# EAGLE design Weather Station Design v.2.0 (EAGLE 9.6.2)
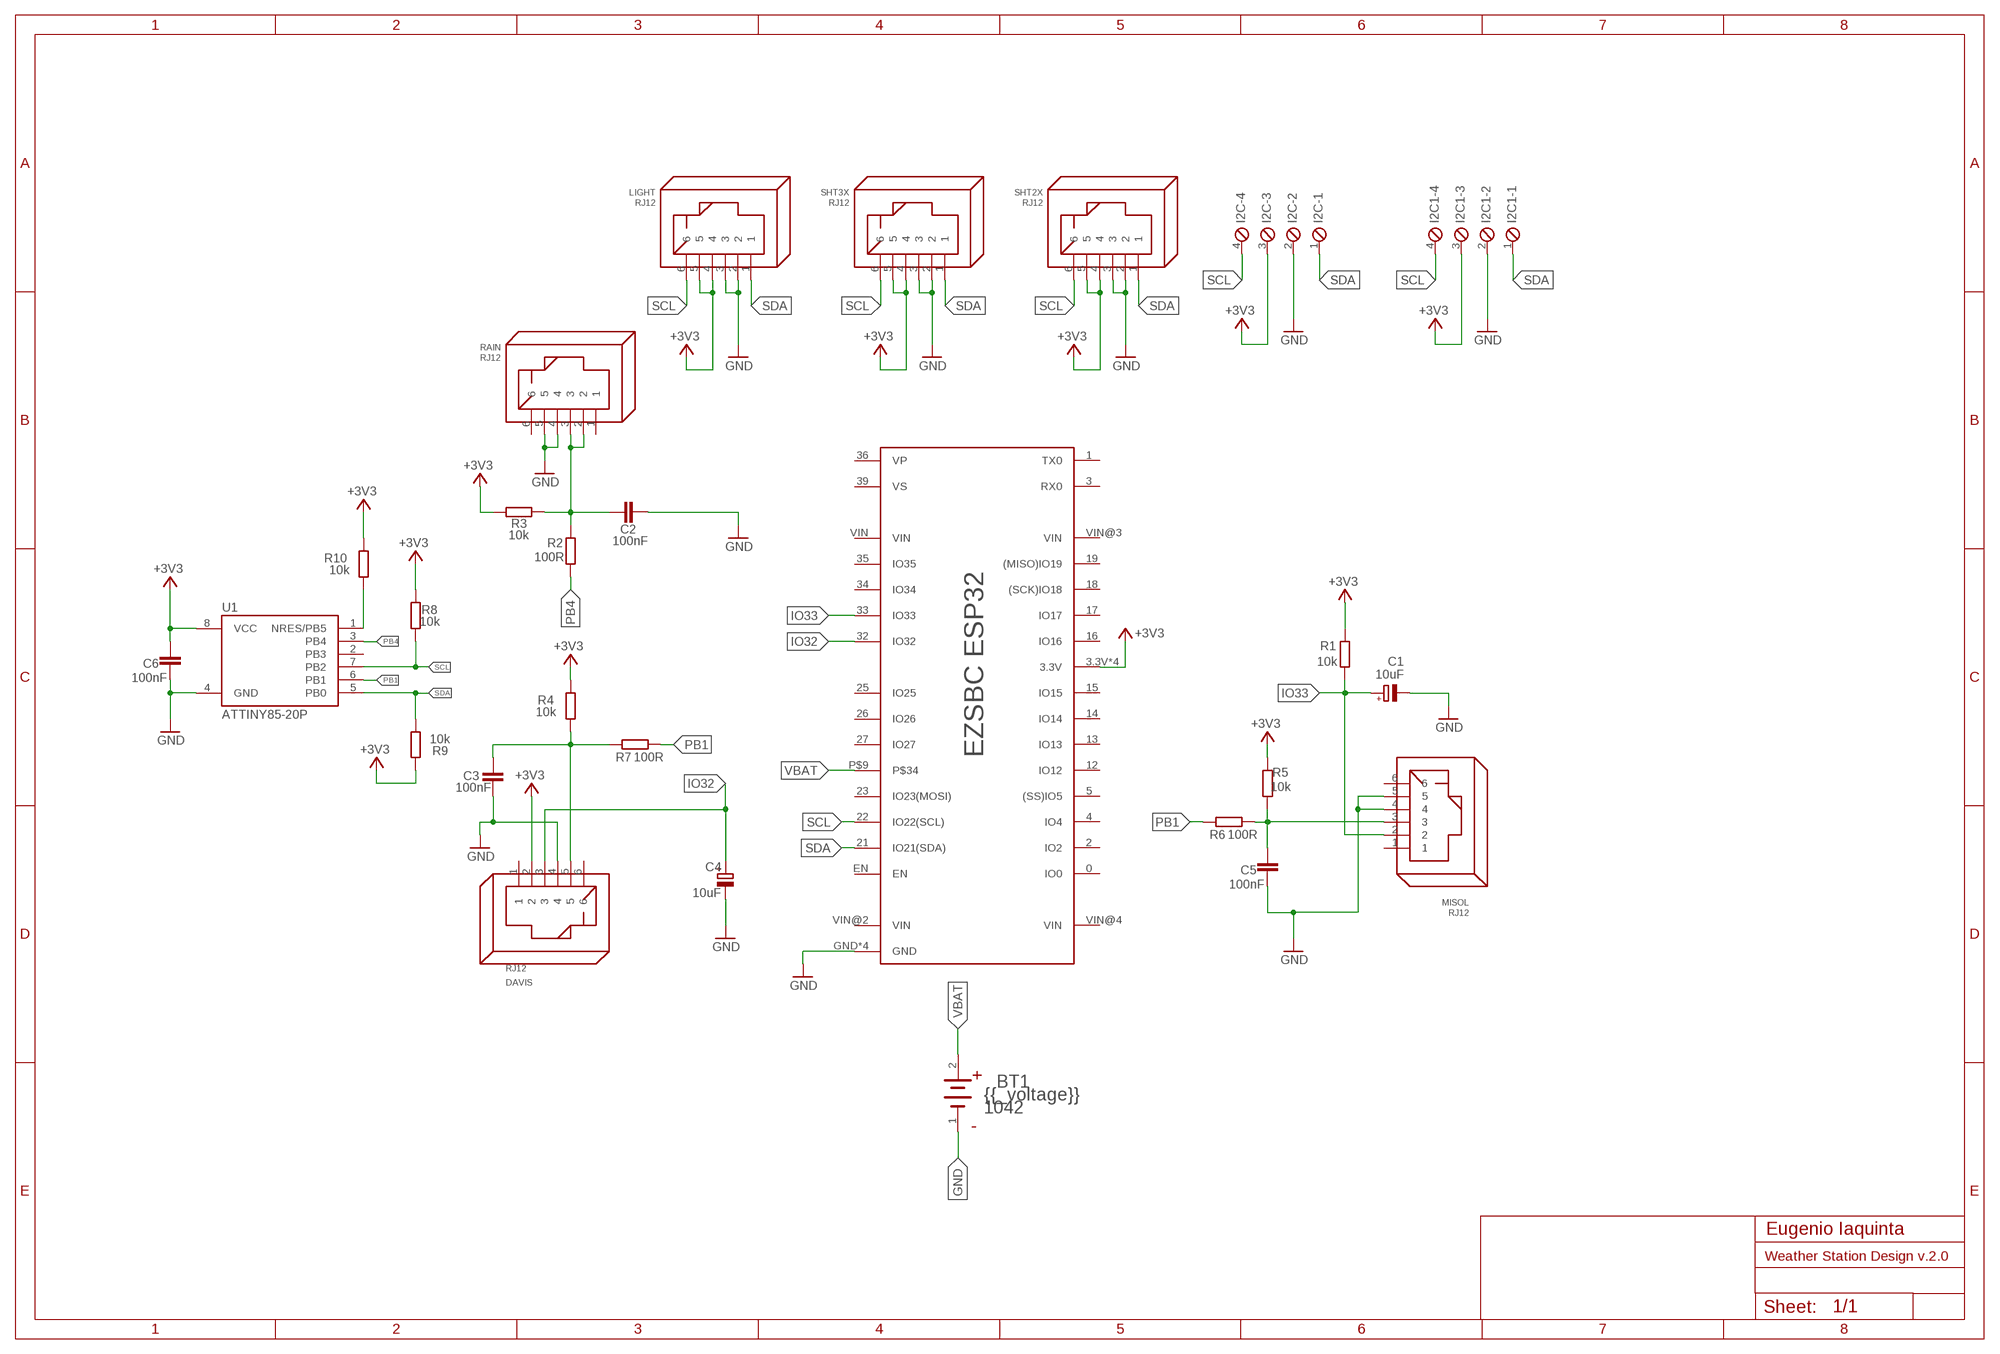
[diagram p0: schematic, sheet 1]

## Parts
BT1  KEYSTONE_1042KEYSTONE_1042_0_0  [KEYSTONE_1042_0]
C1  10uF  CPOL-EUE2.5-5  [E2,5-5]
C2  100nF  C-EUC0805  [C0805]
C3  100nF  C-EUC0805  [C0805]
C4  10uF  CPOL-EUE2.5-5  [E2,5-5]
C5  100nF  C-EUC0805  [C0805]
C6  100nF  C-EUC0805  [C0805]
DAVIS  RJ12  [RJ12]
I2C  MPT4  [4POL254]
I2C1  MPT4  [4POL254]
LIGHT  RJ12  [RJ12]
MISOL  RJ12  [RJ12]
R1  10k  R-EU_M0805  [M0805]
R2  100R  R-EU_M0805  [M0805]
R3  10k  R-EU_M0805  [M0805]
R4  10k  R-EU_M0805  [M0805]
R5  10k  R-EU_M0805  [M0805]
R6  100R  R-EU_M0805  [M0805]
R7  100R  R-EU_M0805  [M0805]
R8  10k  R-EU_M0805  [M0805]
R9  10k  R-EU_M0805  [M0805]
R10  10k  R-EU_M0805  [M0805]
RAIN  RJ12  [RJ12]
SHT2X  RJ12  [RJ12]
SHT3X  RJ12  [RJ12]
U1  ATTINY85-20P  [PDIP08_300MIL]
U$1  EZSBCESP32  [EZSBCBATPRO]

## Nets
+3V3: C6.2 DAVIS.2 I2C1.3 I2C.3 LIGHT.4 LIGHT.5 R1.2 R3.1 R4.2 R5.2 R8.2 R9.2 R10.2 SHT2X.4 SHT2X.5 SHT3X.4 SHT3X.5 U1.8(VCC) U$1.3.3V U$1.3.3V@2(3.3V) U$1.3.3V@4(3.3V) U$1.3.3V@5(3.3V)
GND: BT1.1(CATHODE) C1.- C2.2 C3.2 C4.- C5.1 C6.1 DAVIS.4 I2C1.2 I2C.2 LIGHT.2 LIGHT.3 MISOL.4 MISOL.5 RAIN.4 RAIN.5 SHT2X.2 SHT2X.3 SHT3X.2 SHT3X.3 U1.4(GND) U$1.GND U$1.GND@2(GND) U$1.GND@3(GND) U$1.GND@4(GND)
IO32: C4.+ DAVIS.3 U$1.32(IO32)
IO33: C1.+ MISOL.2 R1.1 U$1.33(IO33)
N$4: C2.1 R2.2 R3.2 RAIN.2 RAIN.3
N$7: R10.1 U1.1(NRES/PB5)
PB1: R6.2 R7.1 U1.6(PB1)
PB4: R2.1 U1.3(PB4)
PIN3: C5.2 MISOL.3 R5.1 R6.1
PIN5: C3.1 DAVIS.5 R4.1 R7.2
SCL: I2C1.4 I2C.4 LIGHT.6 R8.1 SHT2X.6 SHT3X.6 U1.7(PB2) U$1.22(IO22(SCL))
SDA: I2C1.1 I2C.1 LIGHT.1 R9.1 SHT2X.1 SHT3X.1 U1.5(PB0) U$1.21(IO21(SDA))
VBAT: BT1.2(ANODE) U$1.P$9
Unconnected: DAVIS.1 DAVIS.6 MISOL.1 MISOL.6 RAIN.1 RAIN.6 U1.2(PB3) U$1.0(IO0) U$1.1(TX0) U$1.2(IO2) U$1.3(RX0) U$1.4(IO4) U$1.5((SS)IO5) U$1.12(IO12) U$1.13(IO13) U$1.14(IO14) U$1.15(IO15) U$1.16(IO16) U$1.17(IO17) U$1.18((SCK)IO18) U$1.19((MISO)IO19) U$1.23(IO23(MOSI)) U$1.25(IO25) U$1.26(IO26) U$1.27(IO27) U$1.34(IO34) U$1.35(IO35) U$1.36(VP) U$1.39(VS) U$1.EN U$1.VIN U$1.VIN@2(VIN) U$1.VIN@3(VIN) U$1.VIN@4(VIN)

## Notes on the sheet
- Eugenio Iaquinta

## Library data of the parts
BT1 = Keystone - 1042:KEYSTONE_1042: PC BATTERY HOLDER 18650; CENTROID_NOT_SPECIFIED: No; DATASHEET: http://www.keyelco.com/product-pdf.cfm?p=918; DIGIKEY_DESCRIPTION: BATT HOLDER BATTERY 1CELL 18650 SMD; DIGIKEY_PART_NUMBER: 36-1042-ND; IPC_LAND_PATTERN_NAME: CAPC200125X45; LEAD_FREE: yes; MF: Keystone; MOUSER_PART_NUMBER: 534-1042; MPN: 1042; PACKAGE: PTH_BAT_HOLDER_18650; PREFIX: BT; ROHS: yes
C1 C4 = rcl:CPOL-EU: POLARIZED CAPACITOR, European symbol; SPICEPREFIX: C
C2 C3 C5 C6 = rcl:C-EU: CAPACITOR, European symbol; SPICEPREFIX: C
DAVIS LIGHT MISOL RAIN SHT2X SHT3X = con-rj:RJ12: RJ12, RJ14 and RJ25 RJ12, RJ14 and RJ25 jacks side mounted http://www.tycoelectronics.com
I2C I2C1 = con-phoenix-254:MPT4: PHOENIX CONNECTOR; OC_FARNELL: unknown; OC_NEWARK: unknown
R1-R10 = rcl:R-EU_: RESISTOR, European symbol; SPICEPREFIX: R
U1 = attiny25_45_85:ATTINY85*: ATMEL ATtiny 85 Packages: P = PDIP 08 30mil S = SOIC 08 EIAJ 208mil Technologies Note: for complete ordering code (temp. range, finish, tape&reel etc.) see www.atmel.com &bull; Supply Voltage: V = (1.8&hellip;5.5)V | [blank] = (2.7&hellip;5.5)V &bull; Speed: 10 = 10 MHz | 20 = 20 MHz Author: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
U$1 = EzbscBatESP32:EZSBCESP32

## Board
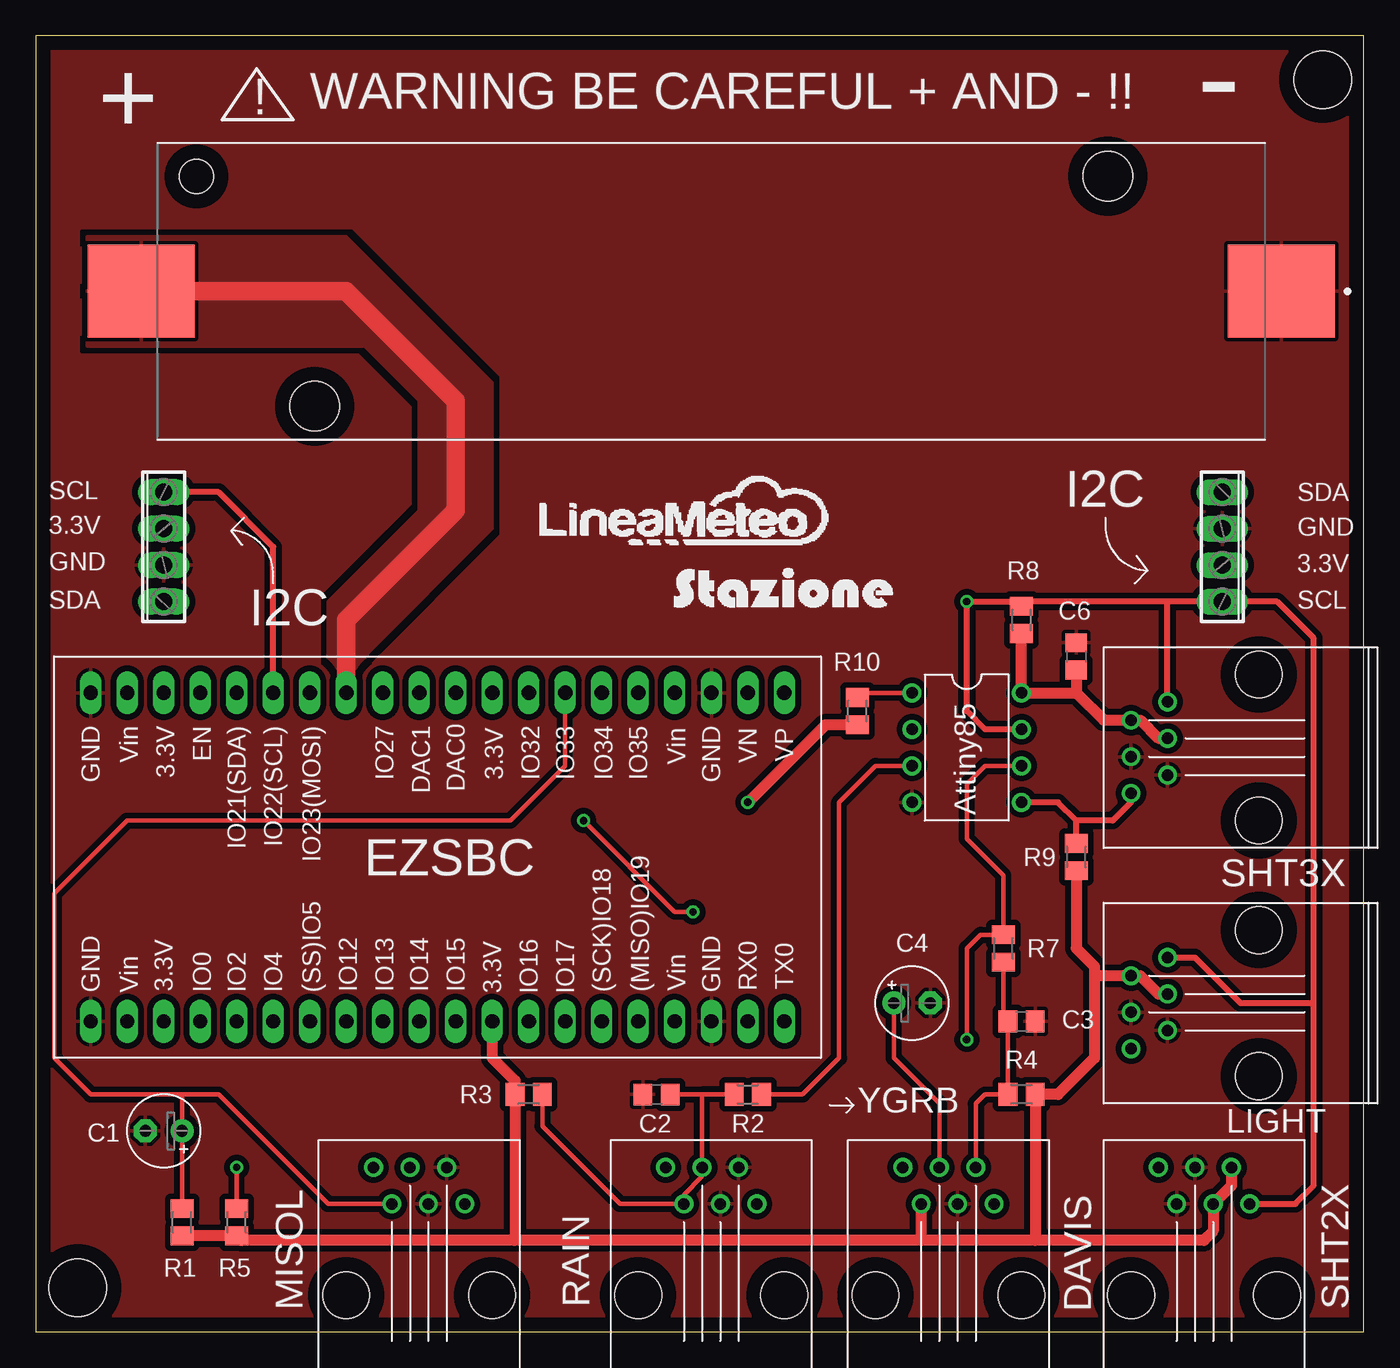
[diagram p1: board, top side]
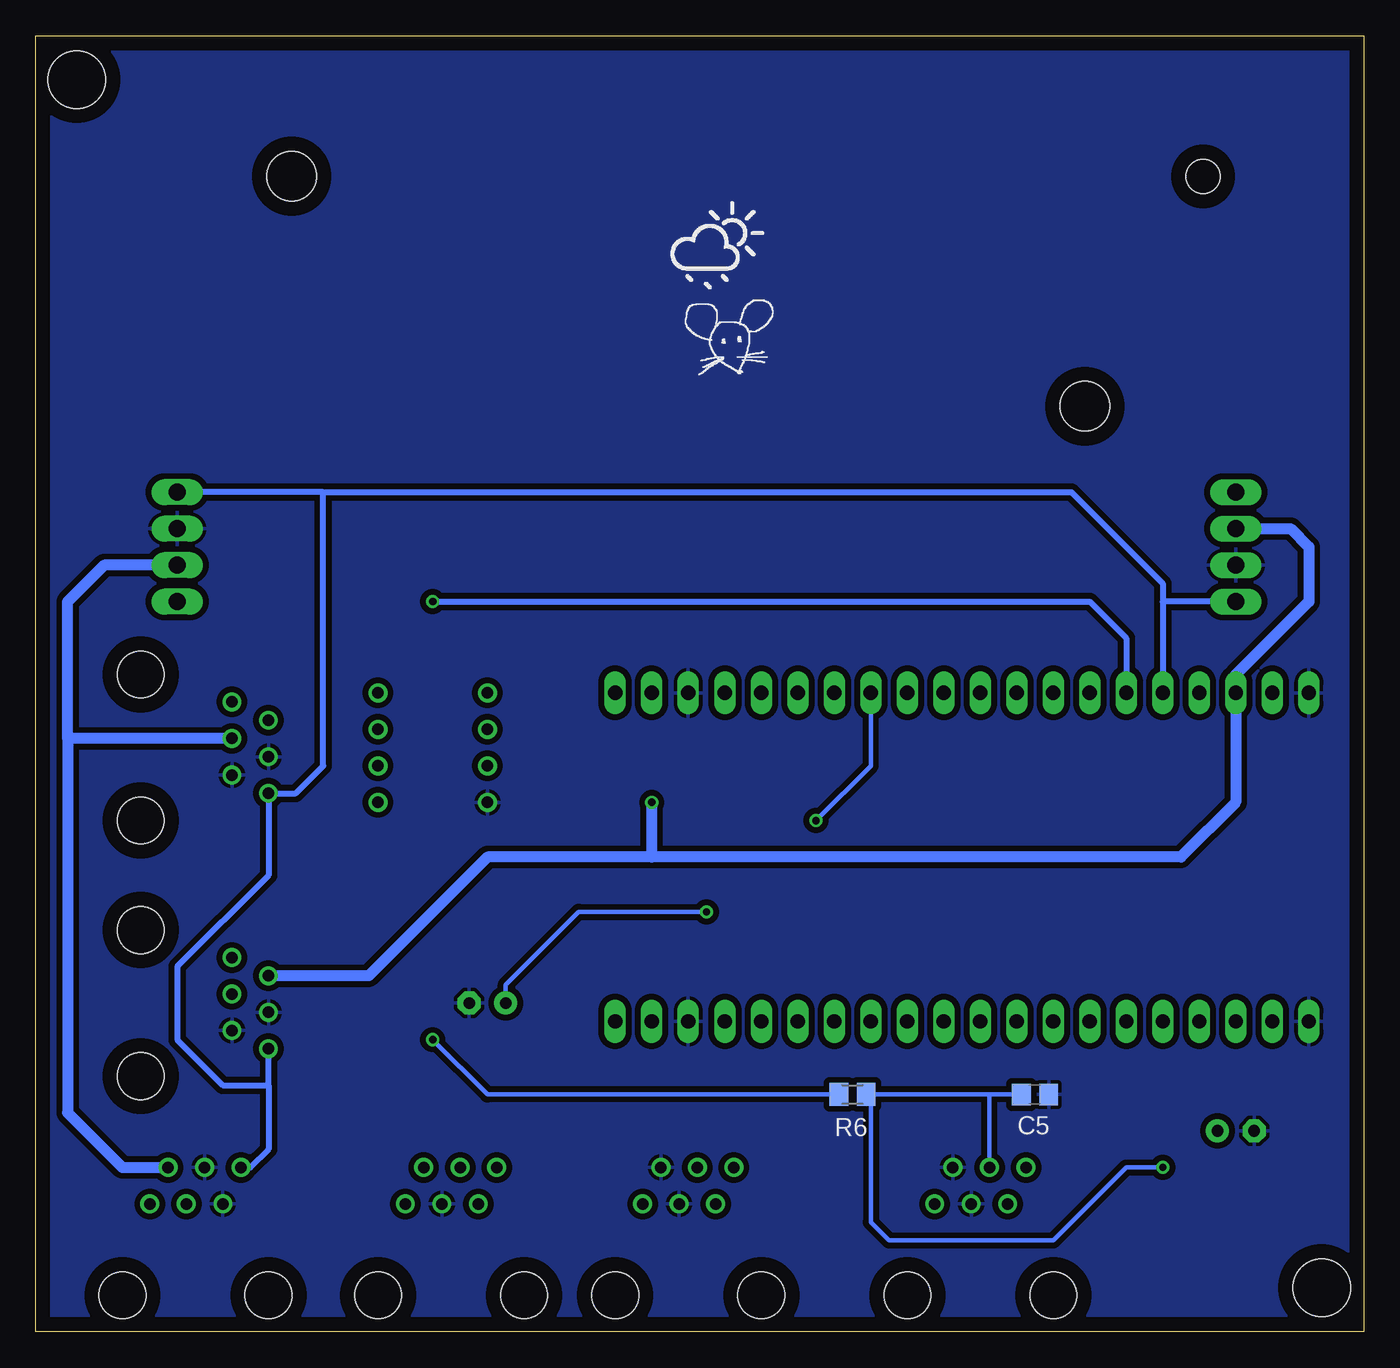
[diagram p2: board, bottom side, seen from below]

Size 92.38 x 90.16 mm. Coordinates in mm from the lower left corner, seen from the top.
Outline: 0,0 92.38,0 92.38,90.16 0,90.16 0,0
Copper layers (1*16): Top 0.035mm / dielectric 1.5mm / Bottom 0.035mm
Design rules "default": minimum track width 6mil, minimum drill 0.35mm, track to track 6mil, track to pad 6mil, pad to pad 6mil, via to via 6mil, smd to smd 6mil, copper to edge 40mil, drill to drill 6mil, minimum pad ring 10mil, minimum via ring 8mil, stop-mask expansion 4mil, vias tented up to drill 0mil, thermal gap 10mil
Holes 4 mm at 89.53,87.12 2.92,3.05

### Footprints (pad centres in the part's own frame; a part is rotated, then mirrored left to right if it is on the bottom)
KEYSTONE_1042_0 = smd 7.46 x 6.47: 1 -39.67,0; 2 39.67,0 | hole 3.45: -27.6,-8; 27.6,8 | hole 2.39: 35.82,-8
E2,5-5 = drill 0.813 pad 1.6: + -1.27,0 | drill 0.813 pad 1.6 octagon: - 1.27,0
C0805 = smd 1.3 x 1.5: 1 -0.95,0; 2 0.95,0
RJ12 = drill 0.8: 1 -8.89,-3.175; 2 -6.35,-1.905; 3 -8.89,-0.635; 4 -6.35,0.635; 5 -8.89,1.905; 6 -6.35,3.175 | hole 3.25: 0,-5.08; 0,5.08
4POL254 = drill 1.2 long: 1 -3.81,0; 2 -1.27,0; 3 1.27,0; 4 3.81,0
M0805 = smd 1.3 x 1.6: 1 -0.95,0; 2 0.95,0
PDIP08_300MIL = drill 0.813: 1 -3.81,-3.81; 2 -1.27,-3.81; 3 1.27,-3.81; 4 3.81,-3.81; 5 3.81,3.81; 6 1.27,3.81; 7 -1.27,3.81; 8 -3.81,3.81
EZSBCBATPRO = drill 1 long: 0 7.62,2.54; 1 7.62,43.18; 2 7.62,5.08; 3 7.62,40.64; 3.3V -15.24,22.86; 3.3V@2 -15.24,0; 3.3V@4 7.62,22.86; 3.3V@5 7.62,0; 4 7.62,7.62; 5 7.62,10.16; 12 7.62,12.7; 13 7.62,15.24; 14 7.62,17.78; 15 7.62,20.32; 16 7.62,25.4; 17 7.62,27.94; 18 7.62,30.48; 19 7.62,33.02; 21 -15.24,5.08; 22 -15.24,7.62; 23 -15.24,10.16; 25 -15.24,20.32; 26 -15.24,17.78; 27 -15.24,15.24; 32 -15.24,25.4; 33 -15.24,27.94; 34 -15.24,30.48; 35 -15.24,33.02; 36 -15.24,43.18; 39 -15.24,40.64; EN -15.24,2.54; GND -15.24,38.1; GND@2 -15.24,-5.08; GND@3 7.62,38.1; GND@4 7.62,-5.08; P$9 -15.24,12.7; VIN -15.24,35.56; VIN@2 -15.24,-2.54; VIN@3 7.62,35.56; VIN@4 7.62,-2.54

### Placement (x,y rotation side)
BT1  46.99,72.39 180 top
C1  8.89,13.97 180 top
C2  43.18,16.51 180 top
C3  68.58,21.59 0 top
C4  60.96,22.86 0 top
C5  22.86,16.51 180 bottom
C6  72.39,46.99 270 top
DAVIS  63.5,2.54 270 top
I2C  82.55,54.61 270 top
I2C1  8.89,54.61 90 top
LIGHT  85.09,22.86 0 top
MISOL  26.67,2.54 270 top
R1  10.16,7.62 270 top
R2  49.53,16.51 180 top
R3  34.29,16.51 0 top
R4  68.58,16.51 0 top
R5  13.97,7.62 270 top
R6  35.56,16.51 180 bottom
R7  67.31,26.67 270 top
R8  68.58,49.53 270 top
R9  72.39,33.02 270 top
R10  57.15,43.18 270 top
RAIN  46.99,2.54 270 top
SHT2X  81.28,2.54 270 top
SHT3X  85.09,40.64 0 top
U1  64.77,40.64 270 top
U$1  8.89,29.21 270 top

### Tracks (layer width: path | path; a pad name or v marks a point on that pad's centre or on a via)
+3V3  (via drill 0.51)
  Top 0.762: SHT2X.5 83.19,10.16 SHT2X.4 81.91,6.99 81.28,6.35 69.53,6.35 | 69.53,6.35 61.59,6.35 | 61.59,6.35 33.27,6.35 | 69.53,6.35 R4.2 71.12,16.51 73.66,19.05 73.66,24.77 | R10.2 54.93,42.23 v49.53,36.83 | R9.2 72.39,26.67 73.66,25.4 73.66,24.77 | 73.66,24.77 LIGHT.5 76.83,24.77 78.11,23.5 LIGHT.4 | 72.39,44.45 U1.8 R8.2 | 72.39,44.45 74.3,42.55 SHT3X.5 76.83,42.55 78.11,41.27 SHT3X.4 | DAVIS.2 61.59,6.35 | R1.2 R5.2 14.29,6.35 33.27,6.35 | 33.27,6.35 33.34,6.42 R3.1 33.34,17.46 31.75,19.05 U$1.3.3V@4 | C6.2 72.39,44.45
  Bottom 0.762: SHT2X.5 86.36,11.43 90.17,15.24 90.17,41.27 | 49.53,33.02 12.7,33.02 8.89,36.83 U$1.3.3V@2 8.89,45.72 3.81,50.8 3.81,54.61 5.08,55.88 I2C1.3 | 49.53,33.02 60.96,33.02 69.22,24.77 LIGHT.5 | I2C.3 87.63,53.34 90.17,50.8 90.17,41.27 | SHT3X.4 90.17,41.27 | v49.53,36.83 49.53,33.02
GND
  pour Top (isolate 0.406, rank 2): 0,0 92.71,0 92.71,90.17 0,90.17
  pour Bottom (isolate 0.406): 0,0 92.71,0 92.71,89.87 0,89.87
IO32  (via drill 0.51)
  Top 0.305: v45.72,29.21 44.45,29.21 v38.1,35.56 | DAVIS.3 62.86,15.88 59.69,19.05 C4.+
  Bottom 0.305: C4.+ 59.69,24.13 54.61,29.21 v45.72,29.21 | v38.1,35.56 34.29,39.37 U$1.32
IO33
  Top 0.305: U$1.33 36.83,39.37 33.02,35.56 6.35,35.56 1.27,30.48 1.27,19.05 3.81,16.51 10.16,16.51 | 10.16,16.51 C1.+ R1.1 | 10.16,16.51 12.7,16.51 20.32,8.89 MISOL.2
N$4
  Top 0.305: C2.1 46.36,16.51 | 46.36,16.51 RAIN.3 46.36,10.79 45.08,9.53 RAIN.2 40.64,8.89 35.24,14.29 R3.2 | R2.2 46.36,16.51
N$7
  Top 0.305: R10.1 57.47,44.45 U1.1
PB1  (via drill 0.51)
  Top 0.305: U1.6 66.04,39.37 64.77,38.1 64.77,34.29 67.31,31.75 R7.1 65.72,27.62 64.77,26.67 v64.77,20.32
  Bottom 0.305: v64.77,20.32 60.96,16.51 R6.2
PB4
  Top 0.305: U1.3 58.42,39.37 55.88,36.83 55.88,19.05 53.34,16.51 R2.1
PIN3  (via drill 0.51)
  Top 0.305: R5.1 v13.97,11.43
  Bottom 0.305: C5.2 26.04,16.51 | 26.04,16.51 R6.1 34.29,16.19 34.29,7.62 33.02,6.35 21.59,6.35 16.51,11.43 v13.97,11.43 | MISOL.3 26.04,16.51
PIN5
  Top 0.305: R7.2 67.31,21.91 C3.1 R4.1 66.04,16.51 65.41,15.88 DAVIS.5
SCL  (via drill 0.51)
  Top 0.406: SHT2X.6 87.63,8.89 88.9,10.16 88.9,22.86 | 88.9,22.86 88.9,48.26 86.36,50.8 I2C.4 78.74,50.8 | SHT3X.6 78.74,50.8 | LIGHT.6 80.64,26.04 83.82,22.86 88.9,22.86 | 78.74,50.8 68.9,50.8 68.74,50.64 | 68.74,50.64 R8.1 | U1.7 66.04,41.91 64.77,43.18 v64.77,50.8 68.58,50.8 68.74,50.64 | U$1.22 16.51,54.61 12.7,58.42 I2C1.4
  Bottom 0.406: v64.77,50.8 19.05,50.8 16.51,48.26 U$1.22
SDA
  Top 0.406: R9.1 72.39,35.56 | 72.39,35.56 71.12,36.83 U1.5 | SHT3X.1 76.2,36.83 74.93,35.56 72.39,35.56
  Bottom 0.406: 13.97,50.8 13.97,52.07 20.32,58.42 72.39,58.42 | 13.97,50.8 U$1.21 | 76.2,17.14 LIGHT.1 | 76.2,17.14 76.2,12.7 77.47,11.43 SHT2X.1 | 72.39,58.42 I2C.1 | 76.2,17.14 79.38,17.14 82.55,20.32 82.55,25.4 76.2,31.75 SHT3X.1 74.3,37.47 72.39,39.37 72.39,58.42 | I2C1.1 13.97,50.8
VBAT
  Top 1.27: U$1.P$9 21.59,49.53 29.21,57.15 29.21,64.77 21.59,72.39 BT1.2
  pour Top (isolate 1.27): 3.56,76.2 21.59,76.2 31.75,66.04 31.75,55.88 22.86,46.99 22.86,43.18 20.32,43.18 20.32,50.8 26.67,57.15 26.67,64.77 22.86,68.58 3.56,68.58

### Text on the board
tPlace: ! | WARNING BE CAREFUL + AND - !! | - | + | SCL | SDA | 3.3V | GND | GND | 3.3V | SDA | SCL | I2C | Attiny85 | YGRB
